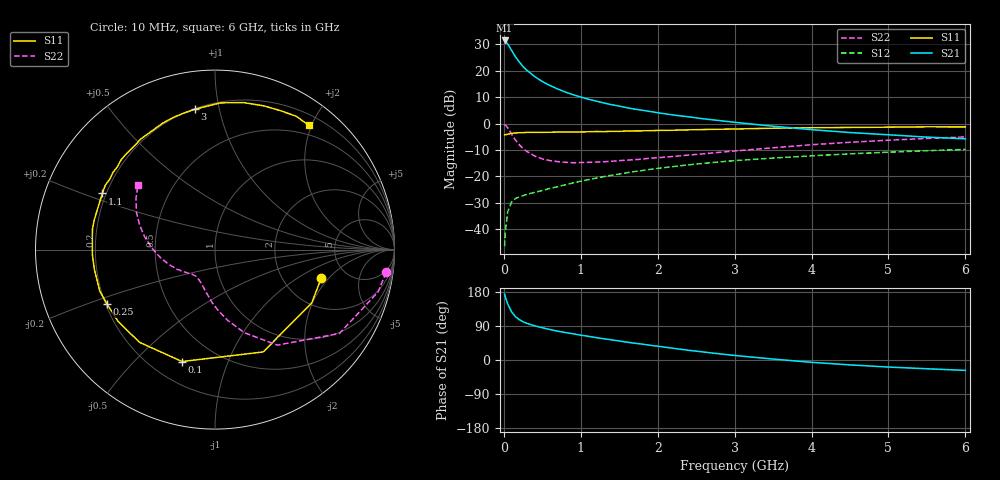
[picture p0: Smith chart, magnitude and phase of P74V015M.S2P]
! SIEMENS Small Signal Semiconductors
! BFP196
! Si NPN RF Bipolar Junction Transistor in SOT143
! VCE = 4 V  IC = 15 mA
! Common Emitter S-Parameters:  May  1996
# GHz  S  MA  R  50
!  f  S11  S21  S12  S22
! GHz  MAG  ANG  MAG  ANG  MAG  ANG  MAG  ANG
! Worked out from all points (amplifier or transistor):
!   36 points, 10 MHz to 6 GHz, reference 50 ohm
!   highest |S21| = 31.5 dB at 10 MHz (marker M1)
!   |S21| within 3 dB of that: start of sweep to 85.14 MHz
!   unconditionally stable (mu >= 1): 770.1 MHz to 3.396 GHz
!   at 250 MHz: K = 0.51, MSG = 24.4 dB, |S12| = -27.3 dB
!   at 1.4 GHz: K = 1.12, MAG = 11.2 dB, |S12| = -19.6 dB
!   at 6 GHz: K = 0.96, MSG = 2.0 dB, |S12| = -9.8 dB
!   S11 on the Smith chart (normalised r, x): 10 MHz: 3.27, -1.65; 100 MHz: 0.32, -0.70; 250 MHz: 0.21, -0.23; 1.1 GHz: 0.19, +0.23; 3 GHz: 0.20, +0.85; 6 GHz: 0.35, +1.96
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0.01  0.613 -14.9  37.38 173.6  0.0048 85.4  0.9618 -7.6
0.02  0.6154 -28.9  36.06 165.8  0.0092 78.5  0.9383 -14.6
0.05  0.6302 -64.8  32.18 148.1  0.0215 63.5  0.8359 -34.0
0.1  0.65 -106.4  24.36 127.2  0.0327 47.9  0.6354 -56.9
0.15  0.6664 -129.2  18.43 114.6  0.0381 41.5  0.4913 -70.5
0.2  0.6717 -143.5  14.7 106.6  0.0411 38.6  0.399 -80.1
0.25  0.6739 -153.4  12 100.8  0.0434 37.6  0.3354 -87.5
0.3  0.6824 -160.3  10.18 96.6  0.0458 38.0  0.2971 -92.9
0.4  0.6811 -170.8  7.779 90.3  0.0501 39.4  0.2439 -101.5
0.5  0.6838 -177.7  6.251 85.2  0.0542 41.8  0.2149 -108.3
0.6  0.6854 175.7  5.237 80.4  0.0596 43.5  0.1993 -113.6
0.7  0.6924 170.3  4.514 76.1  0.064 45.6  0.1906 -117.9
0.8  0.6927 166.2  3.951 72.5  0.0698 46.5  0.1854 -121.7
1.1  0.7011 153.5  2.895 62.4  0.087 48.7  0.185 -129.9
1.3  0.7056 145.9  2.455 56.0  0.0993 48.9  0.1895 -134.7
1.6  0.7238 136.3  1.996 47.1  0.1176 47.9  0.2038 -140.8
2.2  0.7479 118.5  1.455 31.0  0.1538 43.4  0.2388 -152.6
3  0.7901 98.1  1.058 12.0  0.1993 34.9  0.3034 -170.5
3.5  0.8181 87.9  0.891 2.5  0.2231 29.1  0.349 179.1
4.5  0.8458 71.2  0.677 -12.9  0.2677 17.9  0.4429 161.7
5.5  0.8699 58.6  0.555 -23.1  0.307 7.0  0.5239 147.2
6  0.8676 53.0  0.515 -27.4  0.3252 1.1  0.5592 140.3
